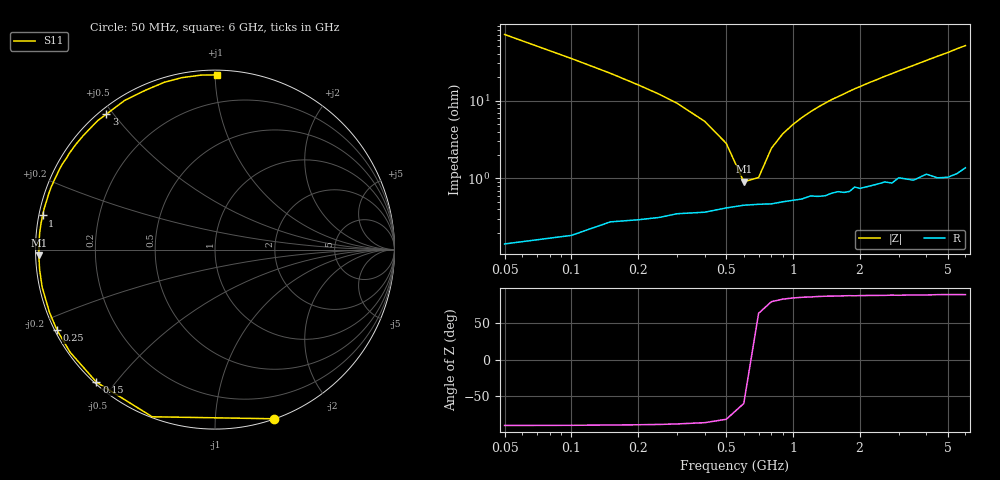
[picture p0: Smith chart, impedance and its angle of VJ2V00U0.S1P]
! Infineon Technologies  Discrete & RF Semiconductors
! BB 914
! Si Tuning Diode in SOT23
! VR = 2 V
! S-Parameters:  July  1999
# GHz  S  MA  R  50
!  f  S11
! GHz  MAG  ANG
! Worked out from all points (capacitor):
!   34 points, 50 MHz to 6 GHz, reference 50 ohm
!   read as one part to ground: C = 44.9 pF near 50 MHz
!   lowest |Z| = 907 mohm at 600 MHz (marker M1)
!   series resonance near 646.2 MHz, so ESL is about 1.4 nH
!   S11 on the Smith chart (normalised r, x): 50 MHz: 0.00, -1.41; 150 MHz: 0.01, -0.45; 250 MHz: 0.01, -0.24; 1 GHz: 0.01, +0.10; 3 GHz: 0.02, +0.48; 6 GHz: 0.03, +1.01
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0.05  0.9981 -70.8
0.1  0.995 -110.6
0.15  0.9908 -131.8
0.2  0.9893 -144.7
0.25  0.9881 -153.0
0.3  0.9864 -159.1
0.4  0.9855 -167.7
0.5  0.9834 -173.6
0.6  0.982 -178.2
0.7  0.9815 177.9
0.8  0.9813 174.5
1  0.9794 168.8
1.3  0.9773 161.3
1.5  0.9754 156.7
1.6  0.9745 154.7
1.7  0.9753 152.7
1.9  0.9716 148.4
2  0.973 146.6
2.2  0.9719 142.7
2.4  0.9707 139.2
2.8  0.9712 132.2
3  0.9673 128.8
3.5  0.9716 121.1
4  0.9686 113.7
4.5  0.974 106.9
5  0.9756 100.9
5.5  0.9754 94.5
6  0.9733 89.3
